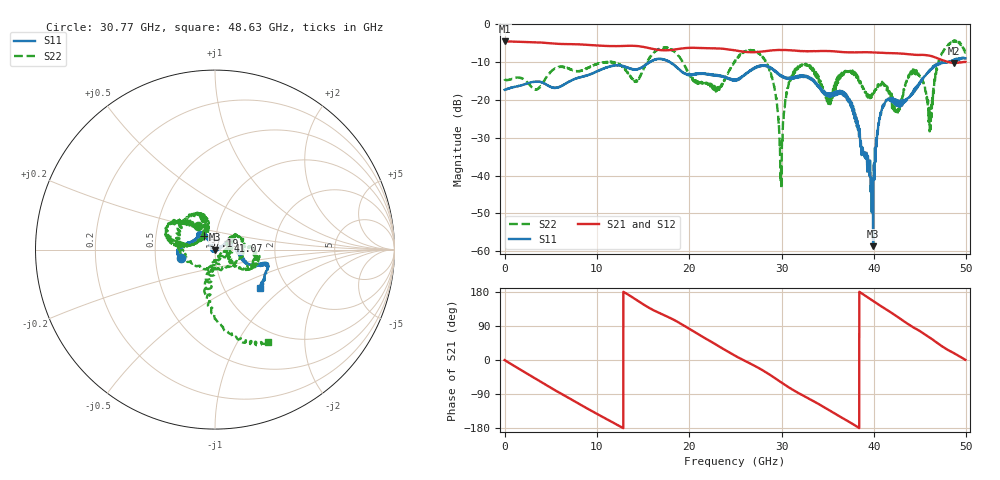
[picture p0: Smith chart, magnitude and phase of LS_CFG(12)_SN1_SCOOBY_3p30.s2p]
!Keysight Technologies,N5245B,MY58422026,A.13.80.08
!Date: Thursday, March 19, 2020 23:30:25
!Correction: S11(Full 2 Port(1,2))
!S21(Full 2 Port(1,2))
!S12(Full 2 Port(1,2))
!S22(Full 2 Port(1,2))
!S2P File: Measurements: S11, S21, S12, S22:
# Hz S DB R 50.0
!freq dBS11 angS11 dBS21 angS21 dBS12 angS12 dBS22 angS22
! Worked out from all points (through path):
!   4991 points, 10 MHz to 49.91 GHz, reference 50 ohm
!   highest |S21| = -4.53 dB at 20 MHz (marker M1); lowest = -10.2 dB at 48.67 GHz (marker M2)
!   group delay of S21, straight-line fit = 39.6 ps
!   lowest |S11| = -58.7 dB at 39.92 GHz (marker M3), VSWR 1.00, Z = 50.1 - j0.0861 ohm
!   |S11| at or under -10 dB: start of sweep to 15.71 GHz; 15.77175 GHz to 15.78643 GHz (14.68 MHz wide, 0.093 % of centre); 17.9 GHz to 48.04 GHz (30.13 GHz wide, 91.4 % of centre)
!   |S22| runs from -43.5 to -4.3 dB; largest |S21 - S12| = 0.0056
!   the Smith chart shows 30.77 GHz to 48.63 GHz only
!   S11 on the Smith chart (normalised r, x): 30.77 GHz: 0.68, -0.06; 37.19 GHz: 0.88, +0.13; 41.07 GHz: 1.16, +0.11; 48.63 GHz: 1.47, -0.70
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1e7  -17.34 -1.5  -4.54 -0.3  -4.52 -0.3  -14.51 0.2
2e7  -17.31 -0.6  -4.53 -0.4  -4.52 -0.4  -14.63 -0.5
8.33e9  -13.99 -76.3  -5.37 -119.3  -5.36 -119.3  -12.27 -86.8
1.665e10  -9.20 -127.9  -6.77 125.2  -6.76 125.3  -6.64 -164.6
2.299e10  -13.65 -143.8  -6.39 39.5  -6.39 39.6  -17.52 -167.8
2.496e10  -14.83 -138.4  -6.90 11.4  -6.88 11.5  -9.83 -174.1
2.835e10  -10.94 -161.1  -7.10 -33.0  -7.10 -32.8  -9.99 -94.0
2.991e10  -13.49 -169.0  -6.83 -58.3  -6.83 -58.1  -41.54 -151.6
3.077e10  -14.13 -166.9  -6.88 -71.9  -6.88 -71.7  -15.81 126.3
3.328e10  -14.44 173.4  -7.13 -106.4  -7.13 -106.1  -11.66 169.2
3.507e10  -18.59 146.6  -7.09 -131.2  -7.03 -130.8  -20.20 138.5
3.719e10  -20.27 128.7  -7.43 -161.4  -7.35 -161.6  -12.47 131.4
3.992e10  -58.68 -47.6  -7.45 155.5  -7.42 155.3  -18.42 -52.2
4.107e10  -21.15 32.0  -7.58 137.5  -7.60 137.4  -16.09 23.2
4.16e10  -19.66 32.9  -7.64 129.4  -7.66 129.2  -17.98 36.8
4.261e10  -20.99 25.6  -7.72 113.1  -7.75 113.0  -22.62 -8.6
4.446e10  -16.83 -7.9  -8.07 83.7  -8.08 83.8  -12.09 -11.0
4.613e10  -12.06 -20.4  -8.38 57.8  -8.40 57.8  -25.69 -43.0
4.711e10  -10.26 -15.5  -9.23 40.8  -9.24 40.8  -9.15 -93.5
4.863e10  -9.63 -40.2  -10.18 18.6  -10.20 18.7  -4.49 -60.1
4.867e10  -9.36 -39.3  -10.23 17.9  -10.24 18.0  -4.36 -57.8
4.991e10  -9.03 -37.9  -9.95 0.3  -9.97 0.2  -7.44 -26.6
